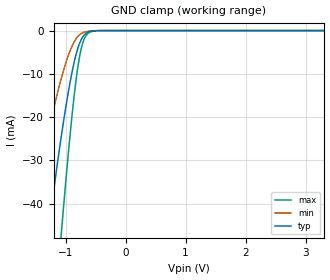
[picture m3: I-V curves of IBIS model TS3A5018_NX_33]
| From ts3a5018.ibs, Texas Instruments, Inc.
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[Model]   TS3A5018_NX_33
Model_type  Terminator
| variable   typ   min   max
C_comp   3.70pF   3.22pF   4.13pF
| C_tri-state   3.70pF   3.22pF   4.13pF
[Temperature Range]   40   100   -40
| Ambient temperature   25   85   -40
[Voltage range]   3.3   3   3.6
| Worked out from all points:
|   GND clamp passes 1 mA (typ) near -0.69 V on its own axis
[GND Clamp]
| TS3A5018_NX_33
|   Voltage   I(typ)   I(min)   I(max)
-3.3V     -364.5mA   -236.4mA   -533.7mA
-1.6V     -85.7mA    -47.27mA   -145.5mA
-1.28V    -46.06mA   -23.24mA   -83.34mA
-1.075V   -24.85mA   -11.27mA   -47.64mA
-1.045V   -22.07mA   -9.782mA   -42.73mA
-955mV    -14.33mA   -5.826mA   -28.63mA
-855mV    -7.237mA   -2.587mA   -14.91mA
-790mV    -3.886mA   -1.292mA   -8.015mA
-725mV    -1.732mA   -584uA     -3.445mA
-630mV    -370.8uA   -175.5uA   -705.3uA
-440mV    -9.98uA    -4.532uA   -23.71uA
3.3V      1.491nA    142.1pA    17.31nA
